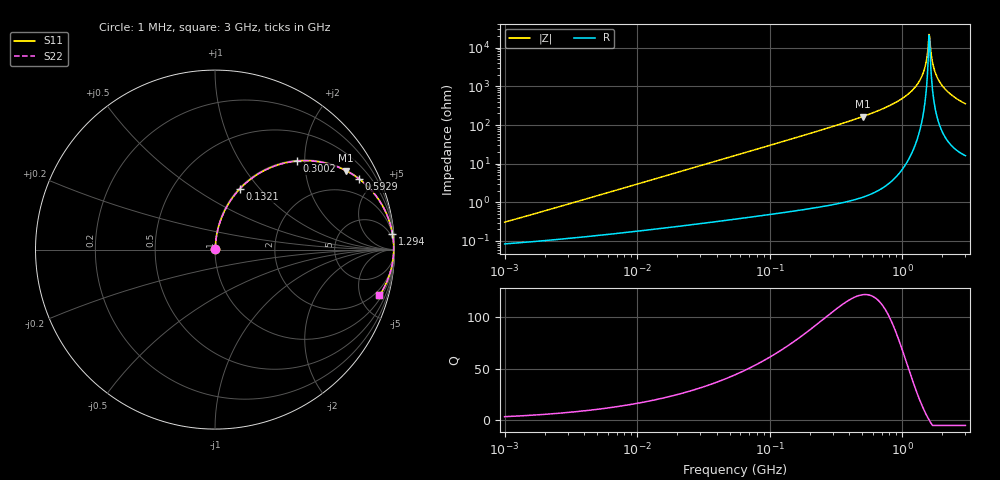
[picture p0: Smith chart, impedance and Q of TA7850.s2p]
# MHz S MA R 50
!Freq  MagS11  AngS11  MagS21  AngS21  MagS12  AngS12  MagS22  AngS22
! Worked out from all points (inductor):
!   801 points, 1 MHz to 3 GHz, reference 50 ohm
!   read as one part in series: L = 47 nH near 1.041 MHz
!   highest Q = 122 at 505.2 MHz (marker M1), where L = 52.2 nH
!   self-resonance near 1.597 GHz
!   S11 on the Smith chart (normalised r, x): 1 MHz: 1.00, +0.01; 132.1 MHz: 1.01, +0.79; 300.2 MHz: 1.02, +1.84; 592.9 MHz: 1.03, +4.06; 1.294 GHz: 2, +22; 3 GHz: 1.32, -7.06
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1  0.003068 74.0  0.9992 -0.2  0.9992 -0.2  0.003068 74.0
3.823119  0.01135 83.0  0.9987 -0.6  0.9987 -0.6  0.01135 83.0
14.47069  0.04266 84.8  0.997 -2.4  0.997 -2.4  0.04266 84.8
54.77226  0.1593 79.5  0.9836 -9.2  0.9836 -9.2  0.1593 79.5
132.1429  0.364 67.9  0.9263 -21.3  0.9263 -21.3  0.364 67.9
209.4008  0.5299 57.4  0.8422 -32.0  0.8422 -32.0  0.5299 57.4
300.2264  0.6735 47.1  0.7329 -42.3  0.7329 -42.3  0.6735 47.1
505.1982  0.853 31.0  0.5149 -58.5  0.5149 -58.5  0.853 31.0
592.9311  0.894 26.1  0.4406 -63.4  0.4406 -63.4  0.894 26.1
792.5923  0.949 17.8  0.3062 -71.6  0.3062 -71.6  0.949 17.8
1059.487  0.9813 10.2  0.1765 -78.9  0.1765 -78.9  0.9813 10.2
1294.266  0.9925 5.2  0.09027 -82.7  0.09027 -82.7  0.9925 5.2
1444.887  0.9952 2.5  0.04371 -82.5  0.04371 -82.5  0.9952 2.5
1503.902  0.9956 1.5  0.02696 -79.9  0.02696 -79.9  0.9956 1.5
1565.327  0.9957 0.6  0.01067 -66.2  0.01067 -66.2  0.9957 0.6
1613.037  0.9956 -0.2  0.005218 32.7  0.005218 32.7  0.9956 -0.2
1645.649  0.9954 -0.6  0.01212 67.5  0.01212 67.5  0.9954 -0.6
1712.864  0.9948 -1.6  0.0285 78.7  0.0285 78.7  0.9948 -1.6
1765.07  0.9942 -2.3  0.04103 80.7  0.04103 80.7  0.9942 -2.3
1950.859  0.9907 -4.8  0.08315 81.2  0.08315 81.2  0.9907 -4.8
2335.937  0.9793 -9.2  0.1599 78.0  0.1599 78.0  0.9793 -9.2
3000  0.951 -15.6  0.269 71.8  0.269 71.8  0.951 -15.6
